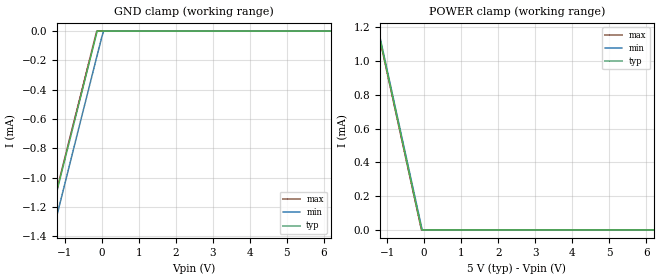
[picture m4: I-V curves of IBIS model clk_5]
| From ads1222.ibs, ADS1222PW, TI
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|   clk_5 Model
[Model]   clk_5
Model_type   Input
Vinl = 1
Vinh = 4
|   typ   min   max
|   (nom PVT)   (fast PVT)   (slow PVT)
|C_comp from frequency sweep method (F= 8MHz)
|Average
C_comp   9.312e-16   7.780e-16   1.116e-15
|C_comp from LC tank measurement(L=1nH)
|Average
|resonant Frequency(Hz)   1.000e+12   1.000e+12   1.000e+12
|C_comp   2.536e-17   2.536e-17   2.536e-17
[Model spec]
Vinl   1   0.9   1.1
Vinh   4   3.6   4.4
| Where nom  PVT is Nominal Process, 5V, 25C
|   Fast PVT is Strong Process,  5.5V, -40C
|   Slow PVT is Weak Process,   4.5V, 85C
[Voltage Range]   5   4.5   5.5
|Ambient Temperature   25   85   -40
|Junction Temperature
[Temperature Range]   25   85   -40
[Power Clamp Reference]   5   4.5   5.5
[GND Clamp Reference]   0   0   0
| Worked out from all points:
|   GND clamp passes 1 mA (typ) near -1.12 V on its own axis
|   POWER clamp passes 1 mA (typ) near -1.06 V on its own axis
[GND Clamp]
|   Voltage   I(typ)   I(min)   I(max)
-5V       -4.998mA   -5.159mA   -4.998mA
-1.728V   -1.621mA   -1.785mA   -1.609mA
-1.25V    -1.136mA   -1.301mA   -1.124mA
-226mV    -105.9uA   -270.6uA   -93.46uA
-138mV    -17.71uA   -182.5uA   -5.421uA
-127mV    -6.705uA   -171.5uA   0A
-115mV    0A         -159.5uA   0A
4mV       0A         -40.57uA   0A
53.5mV    0A         0A         0A
10V       0A         0A         0A
[POWER Clamp]
|   Voltage   I(typ)   I(min)   I(max)
-5V       4.996mA    4.997mA    4.996mA
-1.247V   1.185mA    1.195mA    1.179mA
-1.106V   1.043mA    1.053mA    1.037mA
-72mV     6.562uA    19.92uA    290.4nA
-54.5mV   0A         2.47uA     0A
-45.5mV   0A         0A         0A
10V       0A         0A         0A
